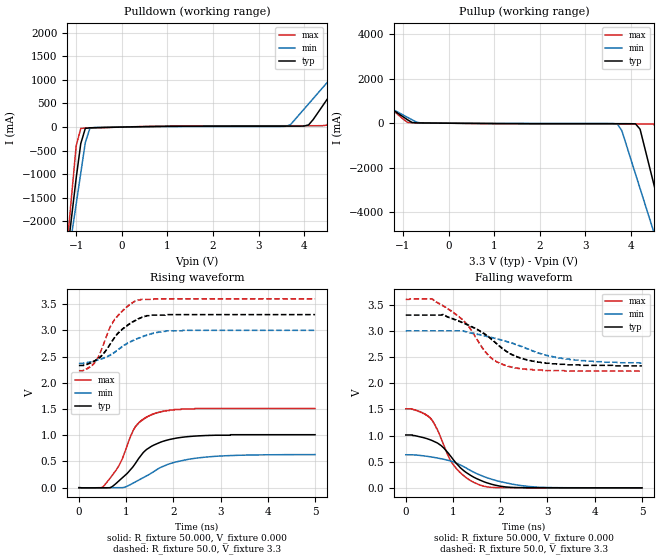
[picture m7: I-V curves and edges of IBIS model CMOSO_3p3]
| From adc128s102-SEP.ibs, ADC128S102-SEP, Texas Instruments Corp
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|   Model CMOSO_3p3
[Model]  CMOSO_3p3
Model_type Output
Enable   Active-High
Vmeas =  1
C_comp   73.44fF   64.02fF   74.18fF
[Temperature Range]   25.000   105.000   -40.000
[Voltage Range]   3.300V   3.0000V   3.600V
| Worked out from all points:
|   slope of the pulldown table from 0 to 0.495 V, typ, clamps not added: 54 ohm
|   slope of the pullup table from 0 to 0.495 V, typ, clamps not added: 60.2 ohm
|   rising waveform, R_fixture 50.000, V_fixture 0.000: 20-80 % time 635ps typ, 888ps min, 471ps max; typ from 0 V to 1.01 V
|   rising waveform, R_fixture 50.0, V_fixture 3.3: 20-80 % time 551ps typ, 744ps min, 456ps max; typ from 2.33 V to 3.3 V
|   falling waveform, R_fixture 50.000, V_fixture 0.000: 20-80 % time 695ps typ, 994ps min, 523ps max; typ from 1.01 V to 0 V
|   falling waveform, R_fixture 50.0, V_fixture 3.3: 20-80 % time 961ps typ, 1.31ns min, 736ps max; typ from 3.3 V to 2.33 V
[Pulldown]
|Voltage   I(typ)   I(min)   I(max)
-3.3V     -19.9A     -16.6A     -24.8A
-1.2V     -2.72A     -2.93A     -2.51A
-1.1V     -1.9A      -2.28A     -1.45A
-1V       -1.08A     -1.63A     -398mA
-900mV    -353mA     -978mA     -27.9mA
-800mV    -27.4mA    -328mA     -22.1mA
-700mV    -15.2mA    -27.3mA    -19.5mA
3.6V      19.8mA     16mA       28.1mA
4.1V      46.7mA     493mA      28.3mA
4.5V      581mA      938mA      40.5mA
5.7V      2.27A      2.28A      2.19A
6.6V      3.53A      3.31A      3.81A
[Pullup]
|Voltage   I(typ)   I(min)   I(max)
-3.3V     3.51A      2.93A      4.32A
-900mV    152mA      262mA      34.4mA
-600mV    12.2mA     10.6mA     16.6mA
3.7V      -21.5mA    -32.9mA    -33mA
3.8V      -21.5mA    -335mA     -33.1mA
4.2V      -269mA     -2.94A     -33.5mA
4.5V      -2.73A     -4.89A     -39.6mA
4.6V      -3.55A     -5.54A     -412mA
4.7V      -4.37A     -6.19A     -1.47A
4.8V      -5.19A     -6.84A     -2.53A
5V        -6.83A     -8.15A     -4.64A
6.6V      -19.9A     -18.5A     -21.5A
[Ramp]
|variable   typ   min   max
dV/dt_r   604.83m/633.2p   378.98m/897.0p   906.49m/475.6p
dV/dt_f   604.80m/694.3p   379.02m/996.1p   906.65m/525.9p
R_load  = 50
[Rising Waveform]
R_fixture = 50.000
V_fixture = 0.000
V_fixture_min = 0.000
V_fixture_max = 0.000
|  time   V(typ)   V(min)   V(max)
0s        63pV       6.35nV     55.6pV
520ps     -1.09mV    -1.71mV    26.3mV
680ps     7.93mV     -1.22mV    203mV
860ps     139mV      -2.07mV    441mV
1.2ns     468mV      112mV      1.17V
1.4ns     703mV      206mV      1.33V
1.61ns    823mV      322mV      1.42V
2.02ns    938mV      483mV      1.49V
2.655ns   994mV      581mV      1.51V
5ns       1.01V      631mV      1.51V
[Rising Waveform]
R_fixture = 50.0
V_fixture = 3.3
V_fixture_min = 3.0
V_fixture_max = 3.6
|  time   V(typ)   V(min)   V(max)
0s        2.33V      2.37V      2.23V
145ps     2.35V      2.38V      2.25V
335ps     2.42V      2.42V      2.38V
520ps     2.55V      2.47V      2.73V
735ps     2.84V      2.57V      3.18V
925ps     3.03V      2.69V      3.37V
1.25ns    3.21V      2.85V      3.58V
1.435ns   3.28V      2.91V      3.59V
1.845ns   3.3V       2.99V      3.6V
5ns       3.3V       3V         3.6V
[Falling Waveform]
R_fixture = 50.000
V_fixture = 0.000
V_fixture_min = 0.000
V_fixture_max = 0.000
|  time   V(typ)   V(min)   V(max)
0s        1.01V      632mV      1.51V
205ps     995mV      628mV      1.49V
505ps     922mV      595mV      1.35V
750ps     807mV      556mV      940mV
1.005ns   541mV      496mV      442mV
1.26ns    306mV      388mV      207mV
1.58ns    143mV      241mV      50.3mV
2.06ns    23.4mV     106mV      2.31mV
2.68ns    1.9mV      20.3mV     741uV
5ns       223uV      533uV      112uV
[Falling Waveform]
R_fixture = 50.0
V_fixture = 3.3
V_fixture_min = 3.0
V_fixture_max = 3.6
|  time   V(typ)   V(min)   V(max)
0s        3.3V       3V         3.6V
560ps     3.3V       3V         3.61V
795ps     3.31V      3V         3.47V
950ps     3.24V      3V         3.39V
1.32ns    3.11V      2.97V      3.1V
1.78ns    2.87V      2.88V      2.5V
2.125ns   2.61V      2.8V       2.33V
2.565ns   2.44V      2.66V      2.26V
3.235ns   2.36V      2.48V      2.24V
5ns       2.33V      2.38V      2.23V
